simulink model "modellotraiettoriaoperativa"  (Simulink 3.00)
settings: Solver=ode45  StartTime=0.0  StopTime=10  RelTol=1e-3
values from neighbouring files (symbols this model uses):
  a = u(9)    [acceler.m]    (also in Dati2lin.m = 1; cin_inversa.m = u(4))
  b1 = 1    [Dati2lin.m]
  b2 = 1    [Dati2lin.m]
  ddsc = 4    [traiettoria1.m]    (also in traiettoria2.m = 2; traiettoria3.m)
  Del1 = 0.0022    [Dati2lin.m]
  Del2 = 0.0022    [Dati2lin.m]
  Dm1 = 0.000172    [Dati2lin.m]
  Dm2 = 0.000071    (= 7.1e-05)    [Dati2lin.m]
  g = u(10)    [acceler.m]    (also in Dati2lin.m = 9.806)
  gom = 1    [traiettoria1.m]    (also in traiettoria2.m; traiettoria3.m; cin_inversa.m = u(3))
  Jm1 = 0.000656    [Dati2lin.m]
  Jm2 = 0.000027    (= 2.7e-05)    [Dati2lin.m]
  kcos = (xf-xi)/sqrt((xf-xi)^2+(yf-yi)^2)    [traiettoria1.m]    (also in traiettoria2.m; traiettoria3.m)
  Kcp1 = 32    [Dati2lin.m]
  Kcp2 = 32    [Dati2lin.m]
  Kcv1 = 0.24275    [Dati2lin.m]
  Kcv2 = 0.029363    [Dati2lin.m]
  Ke1 = 1.43    [Dati2lin.m]
  Ke2 = 0.79    [Dati2lin.m]
  Kel1 = 36.3    [Dati2lin.m]
  Kel2 = 4.6    [Dati2lin.m]
  ksin = (yf-yi)/sqrt((xf-xi)^2+(yf-yi)^2)    [traiettoria1.m]    (also in traiettoria2.m; traiettoria3.m)
  Kt1 = 1.75    [Dati2lin.m]
  Kt2 = 0.97    [Dati2lin.m]
  L1 = 0.060    (= 0.06)    [Dati2lin.m]
  L2 = 0.0438    [Dati2lin.m]
  m1 = u(7)    [acceler.m]    (also in Dati2lin.m = 19)
  m2 = u(8)    [acceler.m]    (also in Dati2lin.m = 9)
  n1 = 100    [Dati2lin.m]
  n2 = 100    [Dati2lin.m]
  q01 = atan2(s1,c1)    [traiettoria1.m]    (also in traiettoria2.m; traiettoria3.m; Dati2lin.m = 0)
  q02 = atan2(s2,c2)    [traiettoria1.m]    (also in traiettoria2.m; traiettoria3.m; Dati2lin.m = 0)
  qm01 = n1*q01 + taulm01/Kel1    [traiettoria1.m]    (also in traiettoria2.m; traiettoria3.m; Dati2lin.m)
  qm02 = n2*q02 + taulm02/Kel2    [traiettoria1.m]    (also in traiettoria2.m; traiettoria3.m; Dati2lin.m)
  R1 = 3.3    [Dati2lin.m]
  R2 = 20.4    [Dati2lin.m]
  tc = dsc/ddsc    (= 0.25)    [traiettoria1.m]    (also in traiettoria2.m = 0.5; traiettoria3.m)
  Tiv1 = 25    [Dati2lin.m]
  Tiv2 = 5.2632    [Dati2lin.m]
  u01 = taulm01/Kt1    [traiettoria1.m]    (also in traiettoria2.m; traiettoria3.m; Dati2lin.m)
  u02 = taulm02/Kt2    [traiettoria1.m]    (also in traiettoria2.m; traiettoria3.m; Dati2lin.m)
  xi = -1.2    [traiettoria1.m]    (also in traiettoria2.m = -1; traiettoria3.m = -1)
  yi = 1    [traiettoria1.m]    (also in traiettoria2.m; traiettoria3.m)

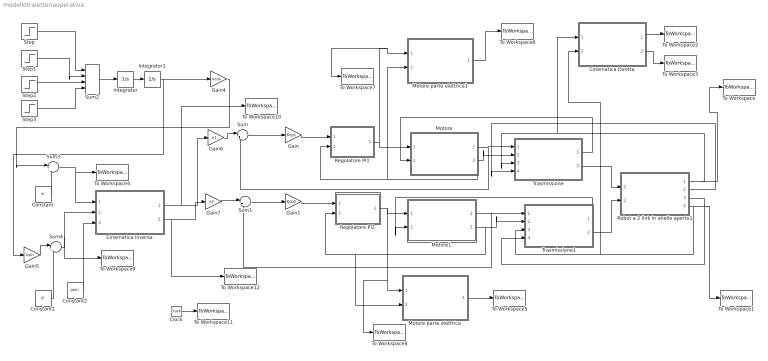
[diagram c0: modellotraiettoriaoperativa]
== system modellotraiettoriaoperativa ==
  Cinematica Diretta : Subsystem  mask(Cinematica diretta di un robot planare a 2 link){a=a}
      mask prompts: a "Lunghezza dei link (a)"
  Cinematica Inversa : Subsystem  mask(Cinematica inversa di un robot planare a 2 link){a=a}
      mask prompts: a "Lunghezza dei link (a)"
  Clock : Clock
  Constant : Constant  Value=xi
  Constant1 : Constant  Value=yi
  Constant2 : Constant  Value=gom
  Gain : Gain  Gain=Kcp1  SaturateOnIntegerOverflow=on
  Gain1 : Gain  Gain=Kcp2  SaturateOnIntegerOverflow=on
  Gain4 : Gain  Gain=kcos  SaturateOnIntegerOverflow=on
  Gain5 : Gain  Gain=ksin  SaturateOnIntegerOverflow=on
  Gain6 : Gain  Gain=n1  SaturateOnIntegerOverflow=on
  Gain7 : Gain  Gain=n2  SaturateOnIntegerOverflow=on
  Integrator : Integrator  ExternalReset=none  InitialConditionSource=internal  InitialCondition=0  LimitOutput=off  UpperSaturationLimit=inf  LowerSaturationLimit=-inf  ShowSaturationPort=off  ShowStatePort=off  AbsoluteTolerance=auto
  Integrator1 : Integrator  ExternalReset=none  InitialConditionSource=internal  InitialCondition=0  LimitOutput=off  UpperSaturationLimit=inf  LowerSaturationLimit=-inf  ShowSaturationPort=off  ShowStatePort=off  AbsoluteTolerance=auto
  Motore : Subsystem  mask(Motore (solo meccanica)){Kt=Kt1, Jm=Jm1, Dm=Dm1, Qm0=qm01}
      mask prompts: Kt "Costante di coppia (Kt)"; Jm "Momento d'inerzia (Jm)"; Dm "Coefficiente di attrito viscoso (Dm)"; Qm0 "Posizione iniziale (Qm0)"
      mask help: Motore controllato in tensione - Modello che tiene conto degli effetti dell'attrito (solo quello viscoso)
  Motore parte elettrica : Subsystem  mask(Motore - parte elettrica){Ke=Ke2, R=R2, L=L2}
      mask prompts: Ke "Costante di forza controelettromotrice (Ke)"; R "Resistenza (R)"; L "Induttanza (L)"
      mask help: Motore - elettrica per calcolare la tensione da imporre ai morsetti, per ottenere corrente necessaria ad attuare il moto desiderato
  Motore parte elettrica1 : Subsystem  mask(Motore - parte elettrica){Ke=Ke1, R=R1, L=L1}
      mask prompts: Ke "Costante di forza controelettromotrice (Ke)"; R "Resistenza (R)"; L "Induttanza (L)"
      mask help: Motore - elettrica per calcolare la tensione da imporre ai morsetti, per ottenere corrente necessaria ad attuare il moto desiderato
  Motore1 : Subsystem  mask(Motore (solo meccanica)){Kt=Kt2, Jm=Jm2, Dm=Dm2, Qm0=qm02}
      mask prompts: Kt "Costante di coppia (Kt)"; Jm "Momento d'inerzia (Jm)"; Dm "Coefficiente di attrito viscoso (Dm)"; Qm0 "Posizione iniziale (Qm0)"
      mask help: Motore controllato in tensione - Modello che tiene conto degli effetti dell'attrito (solo quello viscoso)
  Regolatore PI1 : Subsystem  mask(Controllore PID ISA){Kc=Kcv1, Ti=Tiv1, b=b1, p6=[-inf,inf], u0=u01}
      mask prompts: Kc "Guadagno (Kc)"; Ti "Tempo integrale (Ti)"; b "Peso sul setpoint (b)"; p6 "Saturazione antiwindup ([umin, umax])"; u0 "Variabile di controllo iniziale (u0)"
      mask init:
      | ulow = p6(1);
      | uhigh = p6(2);
  Regolatore PI2 : Subsystem  mask(Controllore PID ISA){Kc=Kcv2, Ti=Tiv2, b=b2, p6=[-inf,inf], u0=u02}
      mask prompts: Kc "Guadagno (Kc)"; Ti "Tempo integrale (Ti)"; b "Peso sul setpoint (b)"; p6 "Saturazione antiwindup ([umin, umax])"; u0 "Variabile di controllo iniziale (u0)"
      mask init:
      | ulow = p6(1);
      | uhigh = p6(2);
  Robot a 2 link in anello aperto1 : Subsystem  mask(Modello del robot planare a 2 link){m1=m1, m2=m2, a=a, q01=q01, q02=q02, g=g}
      mask prompts: m1 "Massa del link 1 (m1)"; m2 "Massa del link 2 (m2)"; a "Lunghezza del link (a)"; q01 "Posizione iniziale link 1 (q01)"; q02 "Posizione iniziale link 2 (q02)"; g "Accelerazione di gravità (g)"
  Step : Step  Time=0  Before=ddsc  After=ddsc  SampleTime=0
  Step1 : Step  Time=tc  Before=0  After=- ddsc  SampleTime=0
  Step2 : Step  Time=tf - tc  Before=0  After=- ddsc  SampleTime=0
  Step3 : Step  Time=tf  Before=0  After=ddsc  SampleTime=0
  Sum : Sum  Inputs=|+-  SaturateOnIntegerOverflow=on
  Sum1 : Sum  Inputs=|+-  SaturateOnIntegerOverflow=on
  Sum2 : Sum  Inputs=|++++  SaturateOnIntegerOverflow=on
  Sum3 : Sum  Inputs=|++  SaturateOnIntegerOverflow=on
  Sum4 : Sum  Inputs=|++  SaturateOnIntegerOverflow=on
  To Workspace : ToWorkspace  VariableName=qout1  SampleTime=-1  SaveFormat=Matrix
  To Workspace1 : ToWorkspace  VariableName=qout2  SampleTime=-1  SaveFormat=Matrix
  To Workspace10 : ToWorkspace  VariableName=qin1  SampleTime=-1  SaveFormat=Matrix
  To Workspace11 : ToWorkspace  VariableName=x  SampleTime=-1  SaveFormat=Matrix
  To Workspace12 : ToWorkspace  VariableName=qin2  SampleTime=-1  SaveFormat=Matrix
  To Workspace2 : ToWorkspace  VariableName=xout  SampleTime=-1  SaveFormat=Matrix
  To Workspace3 : ToWorkspace  VariableName=yout  SampleTime=-1  SaveFormat=Matrix
  To Workspace4 : ToWorkspace  VariableName=xin  SampleTime=-1  SaveFormat=Matrix
  To Workspace5 : ToWorkspace  VariableName=Vm2  SampleTime=-1  SaveFormat=Matrix
  To Workspace6 : ToWorkspace  VariableName=Vm1  SampleTime=-1  SaveFormat=Matrix
  To Workspace7 : ToWorkspace  VariableName=Im1  SampleTime=-1  SaveFormat=Matrix
  To Workspace8 : ToWorkspace  VariableName=Im2  SampleTime=-1  SaveFormat=Matrix
  To Workspace9 : ToWorkspace  VariableName=yin  SampleTime=-1  SaveFormat=Matrix
  Trasmissione : Subsystem  mask(Riduttore){n=n1, Kel=Kel1, Del=Del1}
      mask prompts: n "Rapporto di trasmissione (n)"; Kel "Coefficiente di elasticità (Kel)"; Del "Coefficiente di smorzamento (Del)"
      mask help: Riduttore - Modello che tiene conto dei soli effetti elastici (senza considerare le inerzie, accorpate nel modello del motore) e di un termine di smorzamento
  Trasmissione1 : Subsystem  mask(Riduttore){n=n2, Kel=Kel2, Del=Del2}
      mask prompts: n "Rapporto di trasmissione (n)"; Kel "Coefficiente di elasticità (Kel)"; Del "Coefficiente di smorzamento (Del)"
      mask help: Riduttore - Modello che tiene conto dei soli effetti elastici (senza considerare le inerzie, accorpate nel modello del motore) e di un termine di smorzamento
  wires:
  Sum/1 -> Gain/1
  Sum1/1 -> Gain1/1
  Gain/1 -> Regolatore PI1/1(ysp)
  Gain1/1 -> Regolatore PI2/1(ysp)
  Trasmissione/2("tau_ll ") -> Robot a 2 link in anello aperto1/1(taull1)
  Trasmissione1/2("tau_ll ") -> Robot a 2 link in anello aperto1/2(taull2)
  Trasmissione1/1("tau_lm ") -> Motore1/2(tau_lm)
  Robot a 2 link in anello aperto1/2(dq1) -> Trasmissione/4("dq ")
  Trasmissione/1("tau_lm ") -> Motore/2(tau_lm)
  Motore1/2(dqm) -> Trasmissione1/2(dqm), Regolatore PI2/2(y), Motore parte elettrica/2(dqm)
  Motore/2(dqm) -> Trasmissione/2(dqm), Regolatore PI1/2(y), Motore parte elettrica1/2(dqm)
  Robot a 2 link in anello aperto1/4(q2) -> Trasmissione1/3("q "), Cinematica Diretta/2(q2), To Workspace1/1
  Regolatore PI2/1(u) -> Motore1/1(I), Motore parte elettrica/1(I), To Workspace8/1
  Regolatore PI1/1(u) -> Motore/1(I), Motore parte elettrica1/1(I), To Workspace7/1
  Integrator/1 -> Integrator1/1
  Step/1 -> Sum2/1
  Step2/1 -> Sum2/3
  Step3/1 -> Sum2/4
  Step1/1 -> Sum2/2
  Cinematica Diretta/2(Y) -> To Workspace3/1
  Cinematica Diretta/1(X) -> To Workspace2/1
  Clock/1 -> To Workspace11/1
  Gain6/1 -> Sum/1
  Gain7/1 -> Sum1/1
  Robot a 2 link in anello aperto1/3(dq2) -> Trasmissione1/4("dq ")
  Robot a 2 link in anello aperto1/1(q1) -> Trasmissione/3("q "), Cinematica Diretta/1(q1), To Workspace/1
  Sum2/1 -> Integrator/1
  Integrator1/1 -> Gain4/1, Gain5/1
  Motore parte elettrica1/1(V) -> To Workspace6/1
  Motore/1(qm) -> Trasmissione/1(qm), Sum/2
  Motore1/1(qm) -> Trasmissione1/1(qm), Sum1/2
  Gain4/1 -> Sum3/1
  Gain5/1 -> Sum4/1
  Constant1/1 -> Sum4/2
  Constant/1 -> Sum3/2
  Constant2/1 -> Cinematica Inversa/3(g)
  Sum4/1 -> Cinematica Inversa/2(Y), To Workspace9/1
  Sum3/1 -> Cinematica Inversa/1(X), To Workspace4/1
  Cinematica Inversa/1(q1) -> Gain6/1, To Workspace10/1
  Cinematica Inversa/2(q2) -> Gain7/1, To Workspace12/1
  Motore parte elettrica/1(V) -> To Workspace5/1

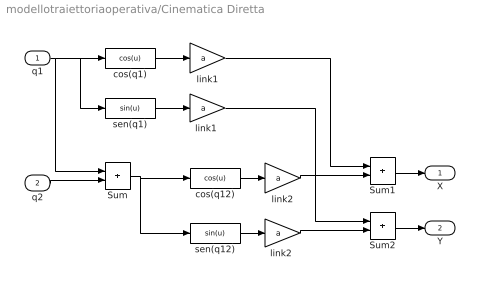
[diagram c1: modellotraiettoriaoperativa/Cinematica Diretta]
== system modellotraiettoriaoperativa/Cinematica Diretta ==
  q1 : Inport  Port=1  PortWidth=-1  SampleTime=-1  DataType=auto
  q2 : Inport  Port=2  PortWidth=-1  SampleTime=-1  DataType=auto
  Sum : Sum  Inputs=++  SaturateOnIntegerOverflow=on
  Sum1 : Sum  Inputs=++  SaturateOnIntegerOverflow=on
  Sum2 : Sum  Inputs=++  SaturateOnIntegerOverflow=on
  cos(q1) : Fcn  Expr=cos(u)
  cos(q12) : Fcn  Expr=cos(u)
  link1 : Gain  Gain=a  SaturateOnIntegerOverflow=on
  "link1 " : Gain  Gain=a  SaturateOnIntegerOverflow=on
  link2 : Gain  Gain=a  SaturateOnIntegerOverflow=on
  "link2 " : Gain  Gain=a  SaturateOnIntegerOverflow=on
  sen(q1) : Fcn  Expr=sin(u)
  sen(q12) : Fcn  Expr=sin(u)
  X : Outport  Port=1
  Y : Outport  Port=2
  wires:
  "link1 "/1 -> Sum2/1
  link1/1 -> Sum1/1
  sen(q12)/1 -> "link2 "/1
  cos(q12)/1 -> link2/1
  Sum/1 -> sen(q12)/1, cos(q12)/1
  sen(q1)/1 -> "link1 "/1
  cos(q1)/1 -> link1/1
  q1/1 -> cos(q1)/1, sen(q1)/1, Sum/1
  q2/1 -> Sum/2
  link2/1 -> Sum1/2
  Sum1/1 -> X/1
  Sum2/1 -> Y/1
  "link2 "/1 -> Sum2/2

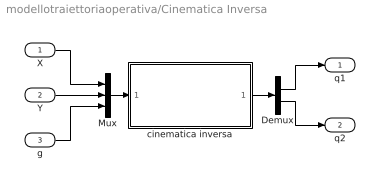
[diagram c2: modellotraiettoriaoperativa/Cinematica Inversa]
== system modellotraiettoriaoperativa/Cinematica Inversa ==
  X : Inport  Port=1  PortWidth=-1  SampleTime=-1  DataType=auto
  Y : Inport  Port=2  PortWidth=-1  SampleTime=-1  DataType=auto
  g : Inport  Port=3  PortWidth=-1  SampleTime=-1  DataType=auto
  Demux : Demux  Outputs=2
  Mux : Mux  Inputs=3
  cinematica inversa : Subsystem
  q1 : Outport  Port=1
  q2 : Outport  Port=2
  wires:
  g/1 -> Mux/3
  X/1 -> Mux/1
  Y/1 -> Mux/2
  Mux/1 -> cinematica inversa/1(u)
  Demux/2 -> q2/1
  Demux/1 -> q1/1
  cinematica inversa/1(y) -> Demux/1

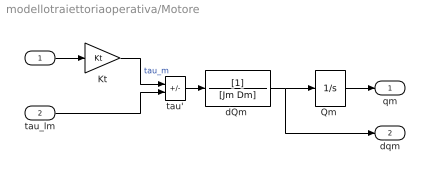
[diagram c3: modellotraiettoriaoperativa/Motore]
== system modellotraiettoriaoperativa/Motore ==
  I : Inport  Port=1  PortWidth=-1  SampleTime=-1  DataType=auto
  tau_lm : Inport  Port=2  PortWidth=-1  SampleTime=-1  DataType=auto
  Kt : Gain  Gain=Kt  SaturateOnIntegerOverflow=on
  "Qm " : Integrator  ExternalReset=none  InitialConditionSource=internal  InitialCondition=Qm0  LimitOutput=off  UpperSaturationLimit=inf  LowerSaturationLimit=-inf  ShowSaturationPort=off  ShowStatePort=off  AbsoluteTolerance=auto
  "dQm " : TransferFcn  Numerator=[1]  Denominator=[Jm Dm]
  tau' : Sum  Inputs=+-  SaturateOnIntegerOverflow=on
  qm : Outport  Port=1
  dqm : Outport  Port=2
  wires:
  "Qm "/1 -> qm/1
  "dQm "/1 -> dqm/1, "Qm "/1
  tau'/1 -> "dQm "/1
  Kt/1 -> tau'/1  "tau_m"
  I/1 -> Kt/1
  tau_lm/1 -> tau'/2

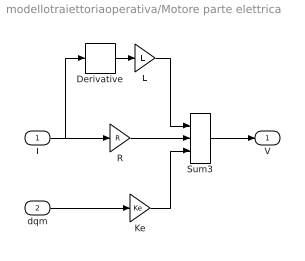
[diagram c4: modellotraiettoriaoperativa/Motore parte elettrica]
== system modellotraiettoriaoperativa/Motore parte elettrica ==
  I : Inport  Port=1  PortWidth=-1  SampleTime=-1  DataType=auto
  dqm : Inport  Port=2  PortWidth=-1  SampleTime=-1  DataType=auto
  Derivative : Derivative
  Ke : Gain  Gain=Ke  SaturateOnIntegerOverflow=on
  L : Gain  Gain=L  SaturateOnIntegerOverflow=on
  R : Gain  Gain=R  SaturateOnIntegerOverflow=on
  Sum3 : Sum  Inputs=+++  SaturateOnIntegerOverflow=on
  V : Outport  Port=1
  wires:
  Sum3/1 -> V/1
  Ke/1 -> Sum3/3
  Derivative/1 -> L/1
  L/1 -> Sum3/1
  I/1 -> Derivative/1, R/1
  R/1 -> Sum3/2
  dqm/1 -> Ke/1

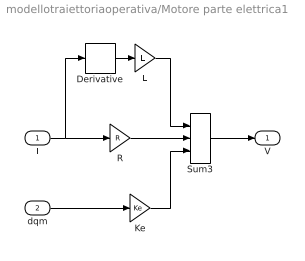
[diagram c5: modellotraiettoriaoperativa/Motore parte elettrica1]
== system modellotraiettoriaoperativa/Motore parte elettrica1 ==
  I : Inport  Port=1  PortWidth=-1  SampleTime=-1  DataType=auto
  dqm : Inport  Port=2  PortWidth=-1  SampleTime=-1  DataType=auto
  Derivative : Derivative
  Ke : Gain  Gain=Ke  SaturateOnIntegerOverflow=on
  L : Gain  Gain=L  SaturateOnIntegerOverflow=on
  R : Gain  Gain=R  SaturateOnIntegerOverflow=on
  Sum3 : Sum  Inputs=+++  SaturateOnIntegerOverflow=on
  V : Outport  Port=1
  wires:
  Sum3/1 -> V/1
  Ke/1 -> Sum3/3
  Derivative/1 -> L/1
  L/1 -> Sum3/1
  I/1 -> Derivative/1, R/1
  R/1 -> Sum3/2
  dqm/1 -> Ke/1

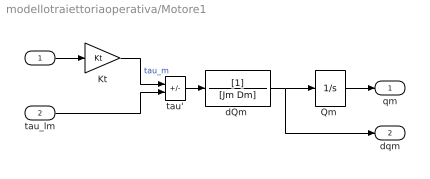
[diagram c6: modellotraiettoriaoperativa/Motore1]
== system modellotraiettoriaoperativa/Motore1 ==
  I : Inport  Port=1  PortWidth=-1  SampleTime=-1  DataType=auto
  tau_lm : Inport  Port=2  PortWidth=-1  SampleTime=-1  DataType=auto
  Kt : Gain  Gain=Kt  SaturateOnIntegerOverflow=on
  "Qm " : Integrator  ExternalReset=none  InitialConditionSource=internal  InitialCondition=Qm0  LimitOutput=off  UpperSaturationLimit=inf  LowerSaturationLimit=-inf  ShowSaturationPort=off  ShowStatePort=off  AbsoluteTolerance=auto
  "dQm " : TransferFcn  Numerator=[1]  Denominator=[Jm Dm]
  tau' : Sum  Inputs=+-  SaturateOnIntegerOverflow=on
  qm : Outport  Port=1
  dqm : Outport  Port=2
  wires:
  "Qm "/1 -> qm/1
  "dQm "/1 -> dqm/1, "Qm "/1
  tau'/1 -> "dQm "/1
  Kt/1 -> tau'/1  "tau_m"
  I/1 -> Kt/1
  tau_lm/1 -> tau'/2

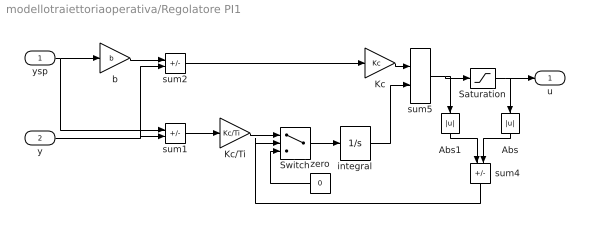
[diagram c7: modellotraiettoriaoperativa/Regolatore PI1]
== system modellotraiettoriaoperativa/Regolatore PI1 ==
  ysp : Inport  Port=1  PortWidth=-1  SampleTime=-1  DataType=auto
  y : Inport  Port=2  PortWidth=-1  SampleTime=-1  DataType=auto
  Abs : Abs  Orientation=down
  Abs1 : Abs  Orientation=down
  Kc : Gain  Gain=Kc  SaturateOnIntegerOverflow=on
  Kc/Ti : Gain  Gain=Kc/Ti  SaturateOnIntegerOverflow=on
  Saturation : Saturate  UpperLimit=uhigh  LowerLimit=ulow
  Switch : Switch  Threshold=0
  b : Gain  Gain=b  SaturateOnIntegerOverflow=on
  integral : Integrator  ExternalReset=none  InitialConditionSource=internal  InitialCondition=u0  LimitOutput=off  UpperSaturationLimit=inf  LowerSaturationLimit=-inf  ShowSaturationPort=off  ShowStatePort=off  AbsoluteTolerance=auto
  sum1 : Sum  Inputs=+-  SaturateOnIntegerOverflow=on
  sum2 : Sum  Inputs=+-  SaturateOnIntegerOverflow=on
  sum4 : Sum  Orientation=down  Inputs=-+  SaturateOnIntegerOverflow=on
  sum5 : Sum  Inputs=++  SaturateOnIntegerOverflow=on
  zero : Constant  Orientation=left  Value=0
  u : Outport  Port=1
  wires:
  integral/1 -> sum5/2
  sum1/1 -> Kc/Ti/1
  Abs/1 -> sum4/2
  Abs1/1 -> sum4/1
  sum5/1 -> Saturation/1, Abs1/1
  Saturation/1 -> Abs/1, u/1
  Switch/1 -> integral/1
  zero/1 -> Switch/3
  sum4/1 -> Switch/2
  Kc/Ti/1 -> Switch/1
  Kc/1 -> sum5/1
  sum2/1 -> Kc/1
  y/1 -> sum1/2, sum2/2
  b/1 -> sum2/1
  ysp/1 -> sum1/1, b/1

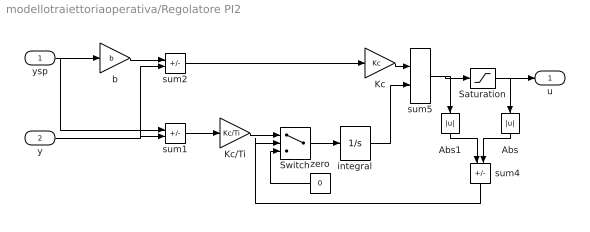
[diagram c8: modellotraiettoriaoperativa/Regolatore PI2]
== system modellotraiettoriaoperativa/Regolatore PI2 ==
  ysp : Inport  Port=1  PortWidth=-1  SampleTime=-1  DataType=auto
  y : Inport  Port=2  PortWidth=-1  SampleTime=-1  DataType=auto
  Abs : Abs  Orientation=down
  Abs1 : Abs  Orientation=down
  Kc : Gain  Gain=Kc  SaturateOnIntegerOverflow=on
  Kc/Ti : Gain  Gain=Kc/Ti  SaturateOnIntegerOverflow=on
  Saturation : Saturate  UpperLimit=uhigh  LowerLimit=ulow
  Switch : Switch  Threshold=0
  b : Gain  Gain=b  SaturateOnIntegerOverflow=on
  integral : Integrator  ExternalReset=none  InitialConditionSource=internal  InitialCondition=u0  LimitOutput=off  UpperSaturationLimit=inf  LowerSaturationLimit=-inf  ShowSaturationPort=off  ShowStatePort=off  AbsoluteTolerance=auto
  sum1 : Sum  Inputs=+-  SaturateOnIntegerOverflow=on
  sum2 : Sum  Inputs=+-  SaturateOnIntegerOverflow=on
  sum4 : Sum  Orientation=down  Inputs=-+  SaturateOnIntegerOverflow=on
  sum5 : Sum  Inputs=++  SaturateOnIntegerOverflow=on
  zero : Constant  Orientation=left  Value=0
  u : Outport  Port=1
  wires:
  integral/1 -> sum5/2
  sum1/1 -> Kc/Ti/1
  Abs/1 -> sum4/2
  Abs1/1 -> sum4/1
  sum5/1 -> Saturation/1, Abs1/1
  Saturation/1 -> Abs/1, u/1
  Switch/1 -> integral/1
  zero/1 -> Switch/3
  sum4/1 -> Switch/2
  Kc/Ti/1 -> Switch/1
  Kc/1 -> sum5/1
  sum2/1 -> Kc/1
  y/1 -> sum1/2, sum2/2
  b/1 -> sum2/1
  ysp/1 -> sum1/1, b/1

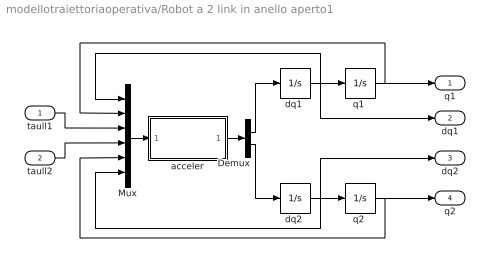
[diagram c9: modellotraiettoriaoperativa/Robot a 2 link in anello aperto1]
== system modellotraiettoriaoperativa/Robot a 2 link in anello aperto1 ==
  taull1 : Inport  Port=1  PortWidth=-1  SampleTime=-1  DataType=auto
  taull2 : Inport  Port=2  PortWidth=-1  SampleTime=-1  DataType=auto
  Demux : Demux  Outputs=2
  Mux : Mux  Inputs=6
  acceler : Subsystem
  "dq1 " : Integrator  ExternalReset=none  InitialConditionSource=internal  InitialCondition=0  LimitOutput=off  UpperSaturationLimit=inf  LowerSaturationLimit=-inf  ShowSaturationPort=off  ShowStatePort=off  AbsoluteTolerance=auto
  "dq2 " : Integrator  ExternalReset=none  InitialConditionSource=internal  InitialCondition=0  LimitOutput=off  UpperSaturationLimit=inf  LowerSaturationLimit=-inf  ShowSaturationPort=off  ShowStatePort=off  AbsoluteTolerance=auto
  "q1 " : Integrator  ExternalReset=none  InitialConditionSource=internal  InitialCondition=q01  LimitOutput=off  UpperSaturationLimit=inf  LowerSaturationLimit=-inf  ShowSaturationPort=off  ShowStatePort=off  AbsoluteTolerance=auto
  "q2 " : Integrator  ExternalReset=none  InitialConditionSource=internal  InitialCondition=q02  LimitOutput=off  UpperSaturationLimit=inf  LowerSaturationLimit=-inf  ShowSaturationPort=off  ShowStatePort=off  AbsoluteTolerance=auto
  q1 : Outport  Port=1
  dq1 : Outport  Port=2
  dq2 : Outport  Port=3
  q2 : Outport  Port=4
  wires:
  taull2/1 -> Mux/4
  taull1/1 -> Mux/3
  Mux/1 -> acceler/1(u)
  Demux/2 -> "dq2 "/1
  Demux/1 -> "dq1 "/1
  acceler/1(y) -> Demux/1
  "q2 "/1 -> Mux/5, q2/1
  "q1 "/1 -> Mux/2, q1/1
  "dq2 "/1 -> Mux/6, dq2/1, "q2 "/1
  "dq1 "/1 -> Mux/1, dq1/1, "q1 "/1

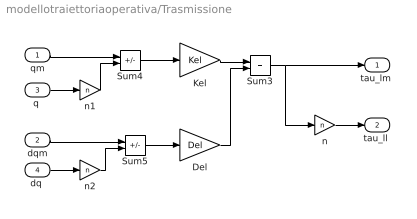
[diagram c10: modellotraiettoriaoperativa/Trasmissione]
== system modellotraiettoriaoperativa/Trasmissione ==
  qm : Inport  Port=1  PortWidth=-1  SampleTime=-1  DataType=auto
  dqm : Inport  Port=2  PortWidth=-1  SampleTime=-1  DataType=auto
  "q " : Inport  Port=3  PortWidth=-1  SampleTime=-1  DataType=auto
  "dq " : Inport  Port=4  PortWidth=-1  SampleTime=-1  DataType=auto
  Del : Gain  Gain=Del  SaturateOnIntegerOverflow=on
  Kel : Gain  Gain=Kel  SaturateOnIntegerOverflow=on
  Sum3 : Sum  Inputs=++  SaturateOnIntegerOverflow=on
  Sum4 : Sum  Inputs=+-  SaturateOnIntegerOverflow=on
  Sum5 : Sum  Inputs=+-  SaturateOnIntegerOverflow=on
  n : Gain  Gain=n  SaturateOnIntegerOverflow=on
  n1 : Gain  Gain=n  SaturateOnIntegerOverflow=on
  n2 : Gain  Gain=n  SaturateOnIntegerOverflow=on
  "tau_lm " : Outport  Port=1
  "tau_ll " : Outport  Port=2
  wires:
  Kel/1 -> Sum3/1
  Sum4/1 -> Kel/1
  n1/1 -> Sum4/2
  qm/1 -> Sum4/1
  Sum3/1 -> "tau_lm "/1, n/1
  Del/1 -> Sum3/2
  Sum5/1 -> Del/1
  n/1 -> "tau_ll "/1
  "q "/1 -> n1/1
  n2/1 -> Sum5/2
  dqm/1 -> Sum5/1
  "dq "/1 -> n2/1

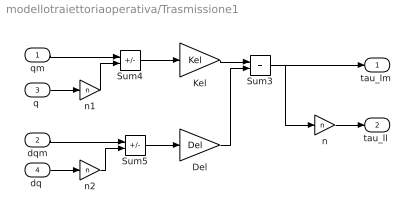
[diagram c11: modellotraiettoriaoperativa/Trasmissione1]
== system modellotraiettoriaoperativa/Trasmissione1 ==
  qm : Inport  Port=1  PortWidth=-1  SampleTime=-1  DataType=auto
  dqm : Inport  Port=2  PortWidth=-1  SampleTime=-1  DataType=auto
  "q " : Inport  Port=3  PortWidth=-1  SampleTime=-1  DataType=auto
  "dq " : Inport  Port=4  PortWidth=-1  SampleTime=-1  DataType=auto
  Del : Gain  Gain=Del  SaturateOnIntegerOverflow=on
  Kel : Gain  Gain=Kel  SaturateOnIntegerOverflow=on
  Sum3 : Sum  Inputs=++  SaturateOnIntegerOverflow=on
  Sum4 : Sum  Inputs=+-  SaturateOnIntegerOverflow=on
  Sum5 : Sum  Inputs=+-  SaturateOnIntegerOverflow=on
  n : Gain  Gain=n  SaturateOnIntegerOverflow=on
  n1 : Gain  Gain=n  SaturateOnIntegerOverflow=on
  n2 : Gain  Gain=n  SaturateOnIntegerOverflow=on
  "tau_lm " : Outport  Port=1
  "tau_ll " : Outport  Port=2
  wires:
  Kel/1 -> Sum3/1
  Sum4/1 -> Kel/1
  n1/1 -> Sum4/2
  qm/1 -> Sum4/1
  Sum3/1 -> "tau_lm "/1, n/1
  Del/1 -> Sum3/2
  Sum5/1 -> Del/1
  n/1 -> "tau_ll "/1
  "q "/1 -> n1/1
  n2/1 -> Sum5/2
  dqm/1 -> Sum5/1
  "dq "/1 -> n2/1

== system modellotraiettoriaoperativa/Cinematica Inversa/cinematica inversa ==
  u : Inport  Port=1  PortWidth=-1  SampleTime=-1  DataType=auto
  Mux : Mux  Inputs=2
  cin_inversa : MATLABFcn  MATLABFcn=cin_inversa  OutputWidth=-1  OutputSignalType=auto
  lunghezza : Constant  Value=a
  y : Outport  Port=1
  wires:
  lunghezza/1 -> Mux/2
  u/1 -> Mux/1
  Mux/1 -> cin_inversa/1
  cin_inversa/1 -> y/1

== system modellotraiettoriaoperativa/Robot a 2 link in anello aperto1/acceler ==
  u : Inport  Port=1  PortWidth=-1  SampleTime=-1  DataType=auto
  MATLAB Fcn : MATLABFcn  MATLABFcn=acceler  OutputWidth=-1  OutputSignalType=auto
  Mux : Mux  Inputs=2
  Parametri : Constant  Value=[m1 m2 a g]'
  y : Outport  Port=1
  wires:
  MATLAB Fcn/1 -> y/1
  Mux/1 -> MATLAB Fcn/1
  u/1 -> Mux/1
  Parametri/1 -> Mux/2
